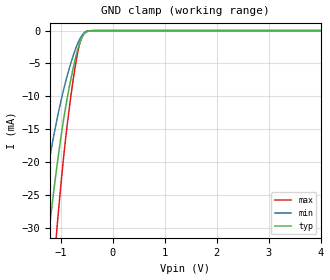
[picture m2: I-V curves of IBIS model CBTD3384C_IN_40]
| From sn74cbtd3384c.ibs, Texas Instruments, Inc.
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[Model]   CBTD3384C_IN_40
Model_type  Input
Vinl=.8
Vinh=2
| variable   typ   min   max
C_comp   4.09pF   2.62pF   6.87pF
[Temperature Range]   40   100   -40
| Ambient temperature   25   85   -40
[Voltage range]   4   4   4
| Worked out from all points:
|   GND clamp passes 1 mA (typ) near -0.59 V on its own axis
[GND Clamp]
| CBTD3384C_IN_40
|   Voltage   I(typ)   I(min)   I(max)
-5V       -417.4mA   -313.8mA   -530.2mA
-1.45V    -47.58mA   -31.24mA   -69.58mA
-1.425V   -45.58mA   -29.9mA    -66.75mA
-1.225V   -30.61mA   -20.02mA   -45.1mA
-1.08V    -21.12mA   -13.88mA   -30.89mA
-925mV    -12.62mA   -8.404mA   -17.9mA
-855mV    -9.459mA   -6.331mA   -13.11mA
-760mV    -5.742mA   -3.855mA   -7.503mA
-695mV    -3.56mA    -2.396mA   -4.286mA
-630mV    -1.831mA   -1.249mA   -1.87mA
-515mV    -268.8uA   -219.5uA   -144.4uA
4V        162.4pA    581.9pA    36.11pA
